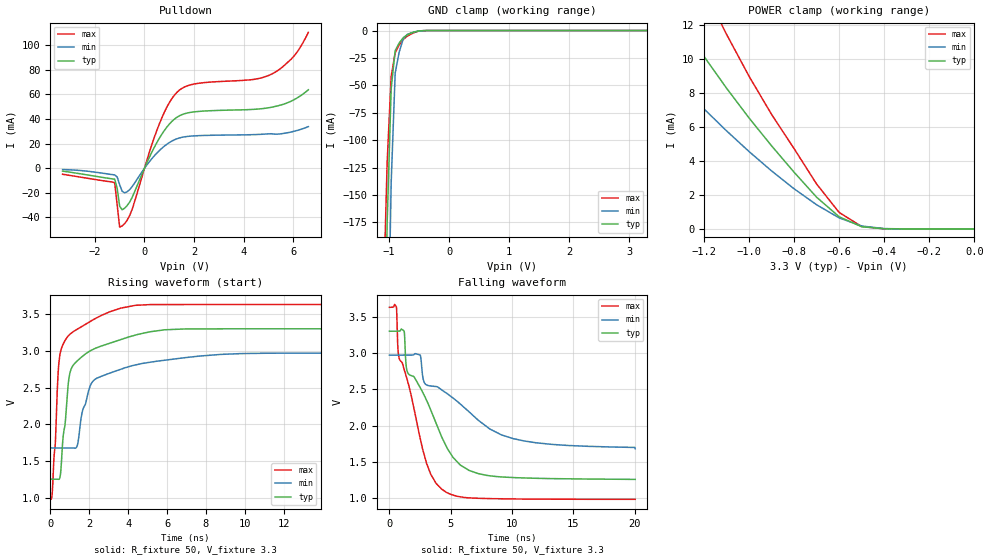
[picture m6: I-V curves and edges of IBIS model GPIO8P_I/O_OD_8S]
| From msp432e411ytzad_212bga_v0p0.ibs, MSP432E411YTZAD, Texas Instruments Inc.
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|   Model Cell GPIO8P_I/O_OD_8S
[Model]   GPIO8P_I/O_OD_8S
Model_type   I/O_open_drain
Polarity   Inverting
Enable   Active-Low
Vinl =  0.8
Vinh =  2
Cref =  15.0000pF
Rref =  100.0000M
Vref =  0V
Vmeas =  1.65
C_comp   5.378567p   4.597605p   6.118031p
[Model Spec]
Vinl   0.8   0.8   0.8
Vinh   2   2   2
[Temperature Range]   25   125   -40
[Voltage Range]   3.3   2.97   3.63
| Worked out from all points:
|   slope of the pulldown table from 0 to 0.495 V, typ, clamps not added: 23.8 ohm
|   GND clamp passes 1 mA (typ) near -0.55 V on its own axis
|   POWER clamp passes 1 mA (typ) near -0.62 V on its own axis
|   rising waveform, R_fixture 50, V_fixture 3.3: 20-80 % time 887ps typ, 1.7ns min, 496ps max; typ from 1.26 V to 3.3 V
|   falling waveform, R_fixture 50, V_fixture 3.3: 20-80 % time 3.46ns typ, 5.66ns min, 2.29ns max; typ from 3.3 V to 1.26 V
| Nom Voltages:
|   VBAT=3.3, VDDC=1.2, VDD=3.3, GND=0
| Min Voltages:
|   VBAT=2.97, VDDC=1.08, VDD=2.97, GND=0
| Max Voltages:
|   VBAT=3.63, VDDC=1.32, VDD=3.63, GND=0
[POWER_clamp]
|   voltage   I(typ)   I(min)   I(max)
-3.3V     116.1mA    496.8mA    244.3mA
-1.533V   17.14mA    11.87mA    23.97mA
-1.3V     12.14mA    8.433mA    16.92mA
-1.267V   11.48mA    7.98mA     15.99mA
-1.133V   8.919mA    6.212mA    12.36mA
-1.1V     8.296mA    5.781mA    11.47mA
-900mV    4.896mA    3.418mA    6.747mA
-800mV    3.341mA    2.365mA    4.729mA
-700mV    1.867mA    1.423mA    2.643mA
-600mV    716.2uA    650.8uA    969.8uA
-500mV    130.1uA    172.8uA    144.6uA
0V        364.7pA    9.133nA    53.42pA
[Pulldown]
|   voltage   I(typ)   I(min)   I(max)
-3.3V     -2.339mA   -1.013mA   -4.845mA
-1.2V     -8.874mA   -5.43mA    -11.86mA
-1.1V     -16.34mA   -7.084mA   -29.69mA
-1V       -30.87mA   -13.32mA   -47.87mA
-900mV    -33.74mA   -18.66mA   -46.85mA
-500mV    -23.82mA   -14.99mA   -33.55mA
600mV     24.46mA    14.43mA    36.18mA
1.3V      41.39mA    23.95mA    61.62mA
2V        45.85mA    26.35mA    68.5mA
5.1V      49.57mA    28.09mA    76.36mA
6V        55.51mA    29.95mA    90.67mA
6.6V      63.82mA    33.88mA    110.5mA
[GND_clamp]
|   voltage   I(typ)   I(min)   I(max)
-3.3V     -16.39A    -15.37A    -17.22A
-1.1V     -384.9mA   -635.5mA   -255.1mA
-1.033V   -175.3mA   -338.1mA   -120.1mA
-966.7mV  -53.11mA   -139.3mA   -41.82mA
-900mV    -18.35mA   -38.91mA   -20.36mA
-833.3mV  -11.36mA   -19.64mA   -13.17mA
-766.7mV  -6.568mA   -7.874mA   -8.128mA
-700mV    -3.981mA   -3.622mA   -5.248mA
-500mV    -326.7uA   -386.2uA   -372.4uA
-366.7mV  -15.8uA    -32.57uA   -14.68uA
3.3V      364.7pA    3.701uA    29.32pA
[Ramp]
| variable   typ   min   max
dV/dt_f   1.24348/3.4450432n 0.78620423/5.623814n   1.6115245/2.2904273n
dV/dt_r  1.2411562/3.2327671n 0.87955263/5.4441898n  1.5983142/2.175063n
R_load = 50
[Rising Waveform]
R_fixture = 50
V_fixture = 3.3
V_fixture_min = 2.97
V_fixture_max = 3.63
|   time   V(typ)   V(min)   V(max)
0s        1.258V     1.681V     983.2mV
105.1ps   1.258V     1.681V     1.08V
395.2ps   1.256V     1.681V     2.667V
527.3ps   1.332V     1.681V     2.992V
1.052ns   2.741V     1.681V     3.236V
1.393ns   2.866V     1.719V     3.296V
2.054ns   3.001V     2.526V     3.4V
2.609ns   3.065V     2.653V     3.48V
8.758ns   3.299V     2.952V     3.63V
20.05ns   3.3V       2.97V      3.63V
[Falling Waveform]
R_fixture = 50
V_fixture = 3.3
V_fixture_min = 2.97
V_fixture_max = 3.63
|   time   V(typ)   V(min)   V(max)
0s        3.3V       2.97V      3.63V
568.9ps   3.3V       2.97V      3.634V
727.9ps   3.3V       2.97V      2.988V
1.199ns   3.302V     2.97V      2.774V
1.476ns   2.733V     2.97V      2.617V
2.517ns   2.52V      2.969V     1.816V
3.029ns   2.348V     2.559V     1.478V
4.236ns   1.854V     2.495V     1.126V
7.209ns   1.339V     2.079V     997.2mV
20.05ns   1.258V     1.681V     982.8mV
